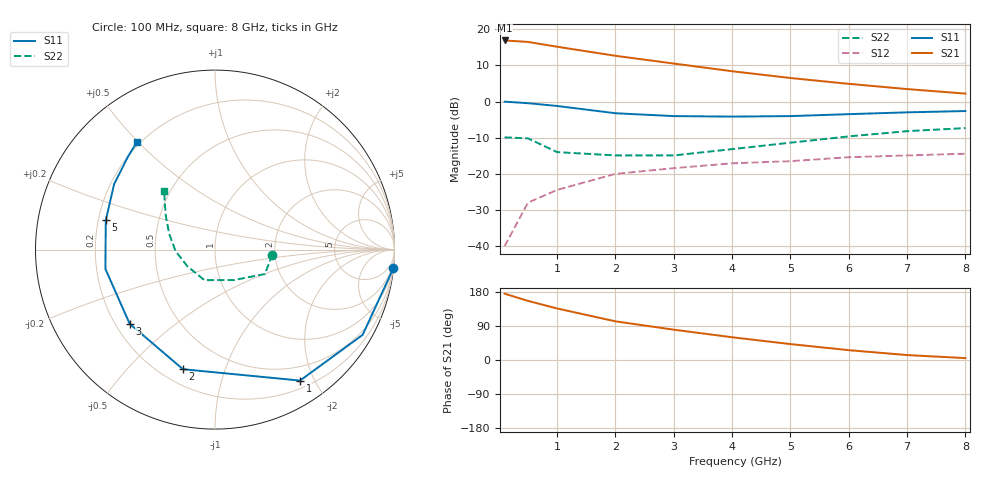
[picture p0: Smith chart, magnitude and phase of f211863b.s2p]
!ATF-21186
!S-PARAMETERS at Vds=3V  Id=70mA.  LAST UPDATED 07-22-92
# ghz s ma r 50
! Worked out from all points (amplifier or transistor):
!   10 points, 100 MHz to 8 GHz, reference 50 ohm
!   highest |S21| = 16.9 dB at 100 MHz (marker M1)
!   |S21| within 3 dB of that: start of sweep to 1.504 GHz
!   unconditionally stable (mu >= 1): 4.333 GHz to end of sweep
!   at 500 MHz: K = 0.22, MSG = 22.2 dB, |S12| = -28.0 dB
!   at 4 GHz: K = 0.96, MSG = 12.7 dB, |S12| = -17.1 dB
!   at 8 GHz: K = 1.05, MAG = 6.9 dB, |S12| = -14.4 dB
!   S11 on the Smith chart (normalised r, x): 100 MHz: 0, -19; 1 GHz: 0.30, -1.80; 2 GHz: 0.29, -0.73; 3 GHz: 0.26, -0.35; 5 GHz: 0.23, +0.12; 8 GHz: 0.19, +0.50
0.1  0.999 -6.0  7.01 175.0  0.01 87.0  0.32 -5.0
0.5  0.95 -30.0  6.69 156.0  0.04 74.0  0.31 -26.0
1  0.87 -57.0  5.74 136.0  0.06 63.0  0.2 -58.0
2  0.69 -105.0  4.3 102.0  0.1 48.0  0.18 -109.0
3  0.63 -139.0  3.36 80.0  0.12 41.0  0.18 -149.0
4  0.62 -170.0  2.63 60.0  0.14 33.0  0.22 -178.0
5  0.63 165.0  2.12 42.0  0.15 28.0  0.27 161.0
6  0.67 147.0  1.76 26.0  0.17 23.0  0.33 146.0
7  0.71 133.0  1.49 13.0  0.18 18.0  0.39 136.0
8  0.74 126.0  1.29 5.0  0.19 16.0  0.43 131.0
